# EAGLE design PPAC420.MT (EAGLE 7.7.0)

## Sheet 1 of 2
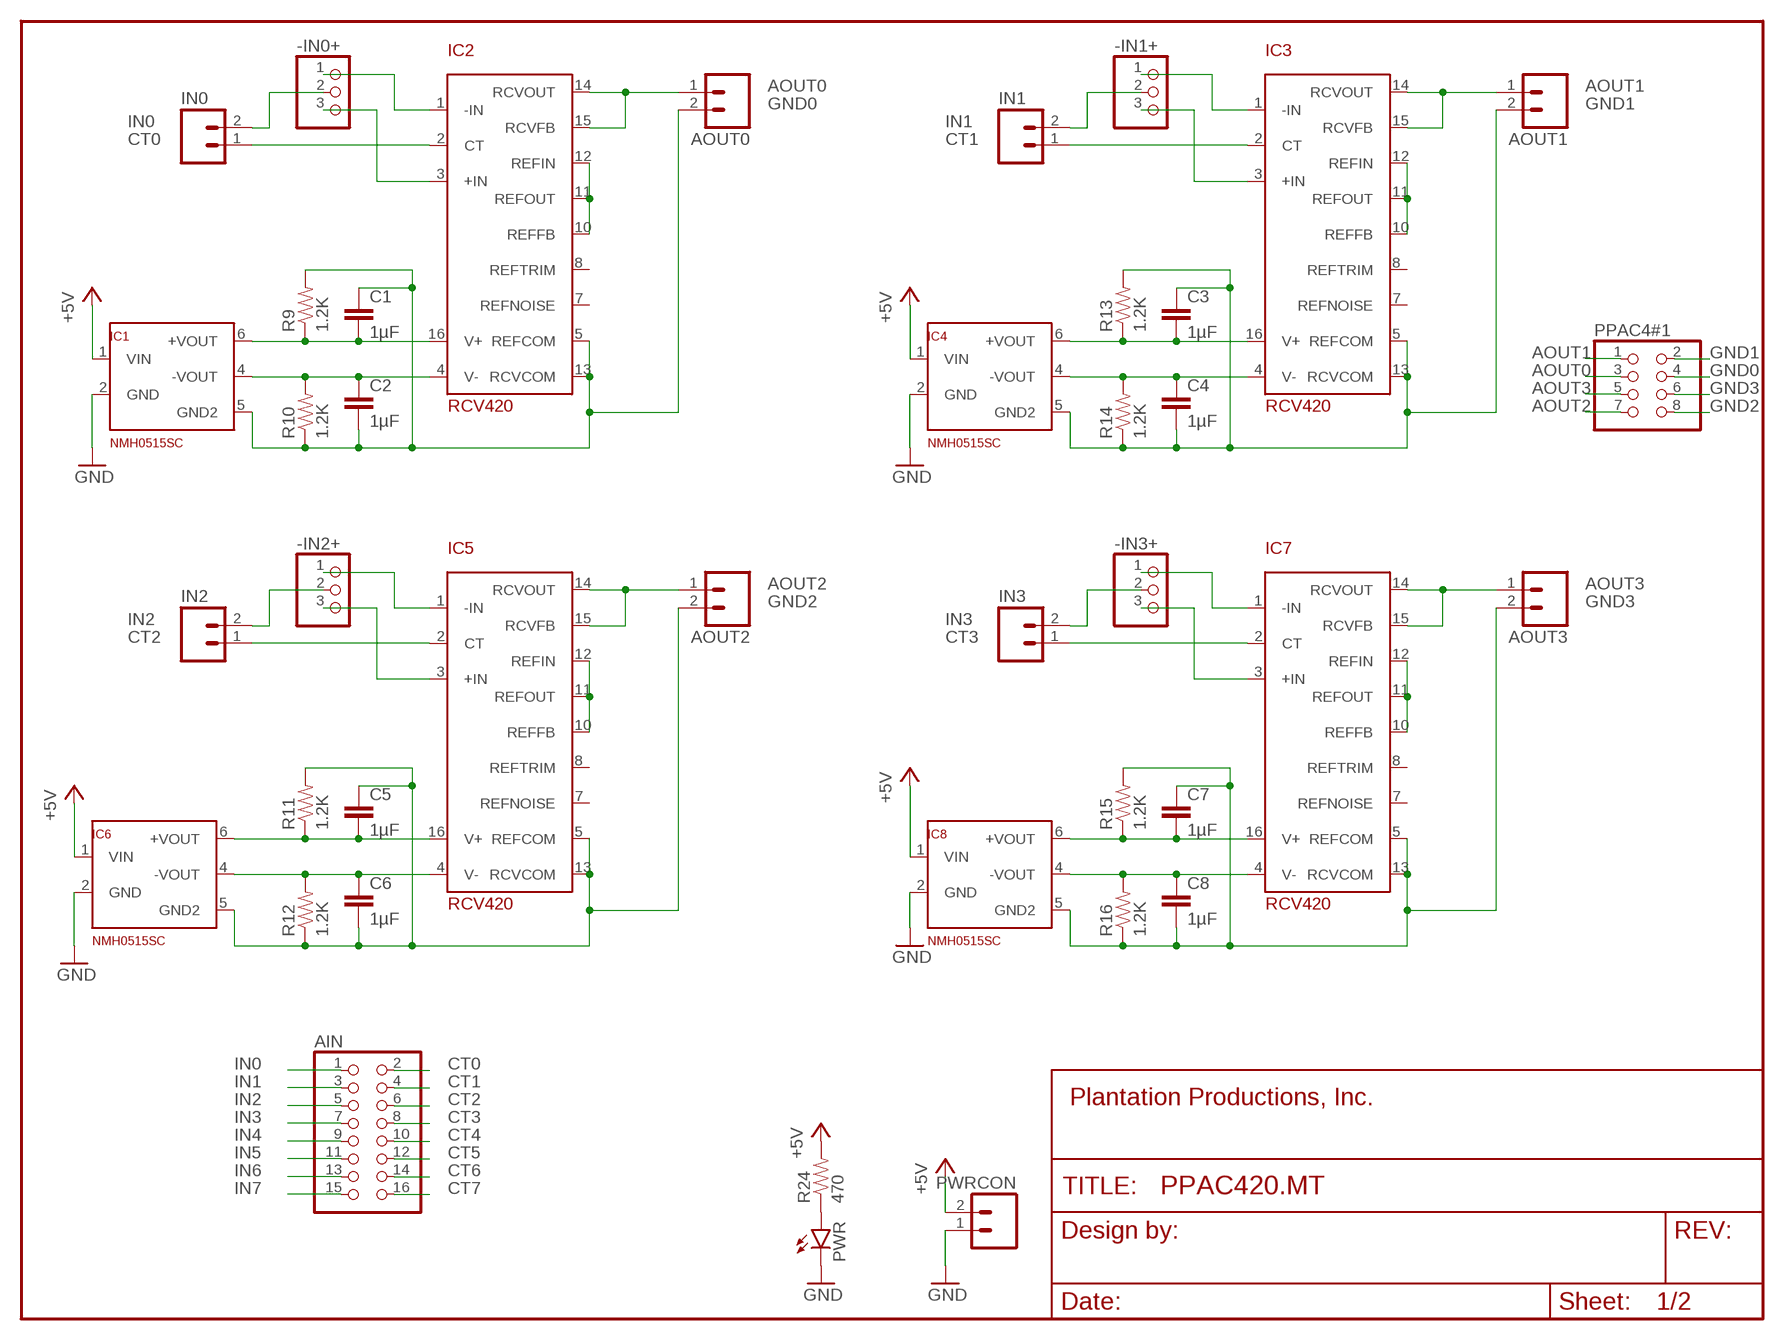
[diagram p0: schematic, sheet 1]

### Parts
-IN0+  PINHD-1X3  [1X03]
-IN1+  PINHD-1X3  [1X03]
-IN2+  PINHD-1X3  [1X03]
-IN3+  PINHD-1X3  [1X03]
AIN  PINHD-2X8  [2X08]
AOUT0  M025MM  [SCREWTERMINAL-5MM-2]
AOUT1  M025MM  [SCREWTERMINAL-5MM-2]
AOUT2  M025MM  [SCREWTERMINAL-5MM-2]
AOUT3  M025MM  [SCREWTERMINAL-5MM-2]
C1  1µF  CAPPTH1  [CAP-PTH-5MM]
C2  1µF  CAPPTH1  [CAP-PTH-5MM]
C3  1µF  CAPPTH1  [CAP-PTH-5MM]
C4  1µF  CAPPTH1  [CAP-PTH-5MM]
C5  1µF  CAPPTH1  [CAP-PTH-5MM]
C6  1µF  CAPPTH1  [CAP-PTH-5MM]
C7  1µF  CAPPTH1  [CAP-PTH-5MM]
C8  1µF  CAPPTH1  [CAP-PTH-5MM]
FRAME4  FRAME-LETTERNO_PACKAGE  [DUMMY]
IC1  NMH0515SC  [SIL6-5A]
IC2  RCV420  [DIL16]
IC3  RCV420  [DIL16]
IC4  NMH0515SC  [SIL6-5A]
IC5  RCV420  [DIL16]
IC6  NMH0515SC  [SIL6-5A]
IC7  RCV420  [DIL16]
IC8  NMH0515SC  [SIL6-5A]
IN0  M025MM  [SCREWTERMINAL-5MM-2]
IN1  M025MM  [SCREWTERMINAL-5MM-2]
IN2  M025MM  [SCREWTERMINAL-5MM-2]
IN3  M025MM  [SCREWTERMINAL-5MM-2]
PPAC4#1  PINHD-2X4  [2X04]
PWR  LED5MM  [LED5MM]
PWRCON  M025MM  [SCREWTERMINAL-5MM-2]
R9  1.2K  1KOHM-1/4W-1%(PTH)  [AXIAL-0.3]
R10  1.2K  1KOHM-1/4W-1%(PTH)  [AXIAL-0.3]
R11  1.2K  1KOHM-1/4W-1%(PTH)  [AXIAL-0.3]
R12  1.2K  1KOHM-1/4W-1%(PTH)  [AXIAL-0.3]
R13  1.2K  1KOHM-1/4W-1%(PTH)  [AXIAL-0.3]
R14  1.2K  1KOHM-1/4W-1%(PTH)  [AXIAL-0.3]
R15  1.2K  1KOHM-1/4W-1%(PTH)  [AXIAL-0.3]
R16  1.2K  1KOHM-1/4W-1%(PTH)  [AXIAL-0.3]
R24  470  1KOHM-1/4W-1%(PTH)  [AXIAL-0.3]

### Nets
+5V: IC1.1(VIN) IC4.1(VIN) IC6.1(VIN) IC8.1(VIN) PWRCON.2 R24.P$2 ; also sheet 2
+15_0: C1.2 IC1.6(+VOUT) IC2.16(V+) R9.P$1
+15_1: C3.2 IC3.16(V+) IC4.6(+VOUT) R13.P$1
+15_2: C5.2 IC5.16(V+) IC6.6(+VOUT) R11.P$1
+15_3: C7.2 IC7.16(V+) IC8.6(+VOUT) R15.P$1
-15_0: C2.1 IC1.4(-VOUT) IC2.4(V-) R10.P$2
-15_1: C4.1 IC3.4(V-) IC4.4(-VOUT) R14.P$2
-15_2: C6.1 IC5.4(V-) IC6.4(-VOUT) R12.P$2
-15_3: C8.1 IC7.4(V-) IC8.4(-VOUT) R16.P$2
AOUT0: AOUT0.1 IC2.14(RCVOUT) IC2.15(RCVFB) PPAC4#1.3
AOUT1: AOUT1.1 IC3.14(RCVOUT) IC3.15(RCVFB) PPAC4#1.1
AOUT2: AOUT2.1 IC5.14(RCVOUT) IC5.15(RCVFB) PPAC4#1.7
AOUT3: AOUT3.1 IC7.14(RCVOUT) IC7.15(RCVFB) PPAC4#1.5
CT0: AIN.2 IC2.2(CT) IN0.1
CT1: AIN.4 IC3.2(CT) IN1.1
CT2: AIN.6 IC5.2(CT) IN2.1
CT3: AIN.8 IC7.2(CT) IN3.1
CT4: AIN.10 ; also sheet 2
CT5: AIN.12 ; also sheet 2
CT6: AIN.14 ; also sheet 2
CT7: AIN.16 ; also sheet 2
GND [Ground]: IC1.2(GND) IC4.2(GND) IC6.2(GND) IC8.2(GND) PWR.K(C) PWRCON.1 ; also sheet 2
GND0 [Ground]: AOUT0.2 C1.1 C2.2 IC1.5(GND2) IC2.5(REFCOM) IC2.13(RCVCOM) PPAC4#1.4 R9.P$2 R10.P$1
GND1: AOUT1.2 C3.1 C4.2 IC3.5(REFCOM) IC3.13(RCVCOM) IC4.5(GND2) PPAC4#1.2 R13.P$2 R14.P$1
GND2: AOUT2.2 C5.1 C6.2 IC5.5(REFCOM) IC5.13(RCVCOM) IC6.5(GND2) PPAC4#1.8 R11.P$2 R12.P$1
GND3: AOUT3.2 C7.1 C8.2 IC7.5(REFCOM) IC7.13(RCVCOM) IC8.5(GND2) PPAC4#1.6 R15.P$2 R16.P$1
IN0: -IN0+.2 AIN.1 IN0.2
IN1: -IN1+.2 AIN.3 IN1.2
IN2: -IN2+.2 AIN.5 IN2.2
IN3: -IN3+.2 AIN.7 IN3.2
IN4: AIN.9 ; also sheet 2
IN5: AIN.11 ; also sheet 2
IN6: AIN.13 ; also sheet 2
IN7: AIN.15 ; also sheet 2
N$3: IC2.10(REFFB) IC2.11(REFOUT) IC2.12(REFIN)
N$4: IC3.10(REFFB) IC3.11(REFOUT) IC3.12(REFIN)
N$7: IC5.10(REFFB) IC5.11(REFOUT) IC5.12(REFIN)
N$10: IC7.10(REFFB) IC7.11(REFOUT) IC7.12(REFIN)
N$25: -IN1+.1 IC3.1(-IN)
N$26: -IN1+.3 IC3.3(+IN)
N$27: -IN0+.1 IC2.1(-IN)
N$28: -IN0+.3 IC2.3(+IN)
N$29: -IN2+.1 IC5.1(-IN)
N$30: -IN2+.3 IC5.3(+IN)
N$31: -IN3+.1 IC7.1(-IN)
N$32: -IN3+.3 IC7.3(+IN)
N$41: PWR.A R24.P$1
Unconnected: IC2.6(NCA) IC2.7(REFNOISE) IC2.8(REFTRIM) IC2.9(NCB) IC3.6(NCA) IC3.7(REFNOISE) IC3.8(REFTRIM) IC3.9(NCB) IC5.6(NCA) IC5.7(REFNOISE) IC5.8(REFTRIM) IC5.9(NCB) IC7.6(NCA) IC7.7(REFNOISE) IC7.8(REFTRIM) IC7.9(NCB)

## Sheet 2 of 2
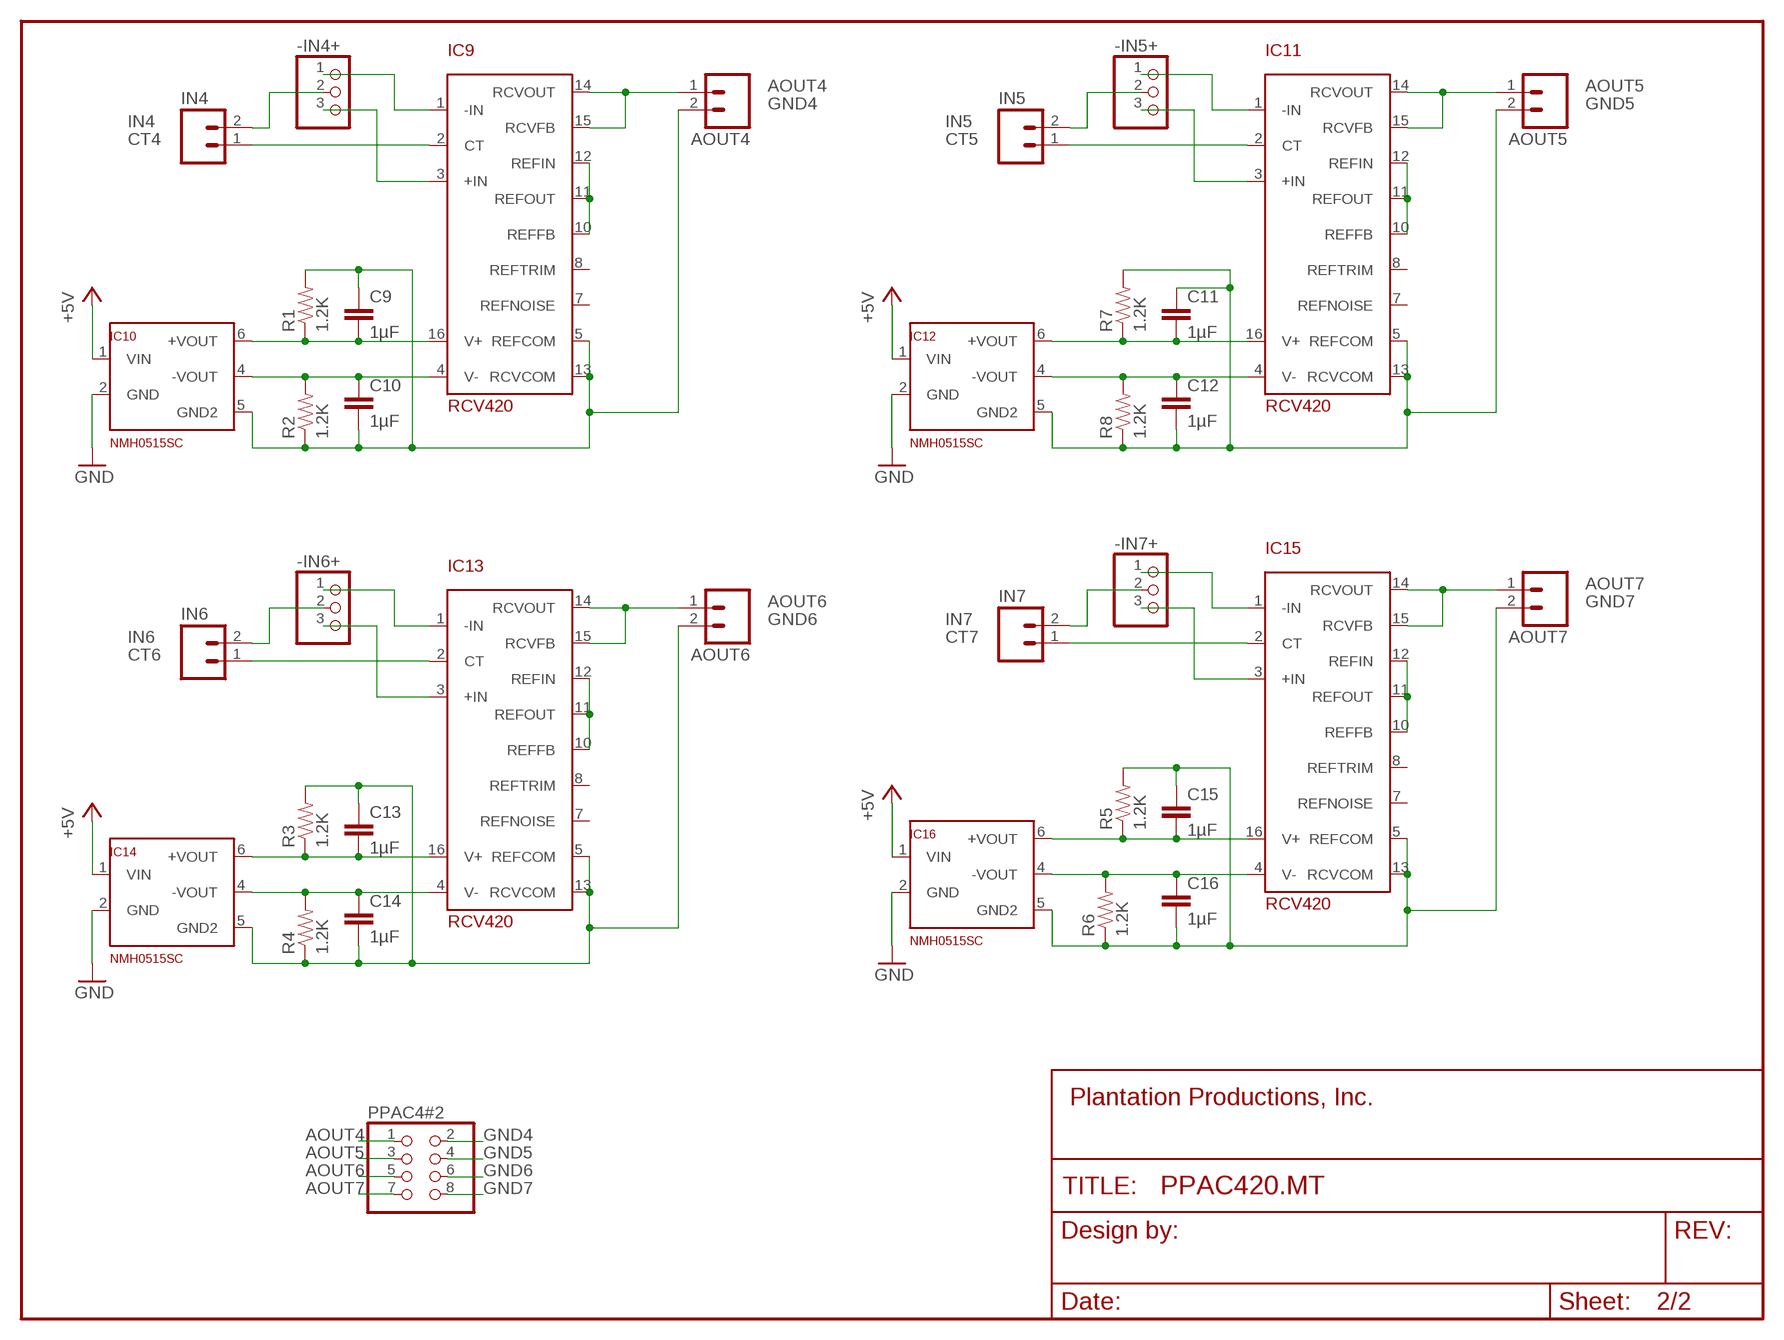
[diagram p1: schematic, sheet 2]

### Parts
-IN4+  PINHD-1X3  [1X03]
-IN5+  PINHD-1X3  [1X03]
-IN6+  PINHD-1X3  [1X03]
-IN7+  PINHD-1X3  [1X03]
AOUT4  M025MM  [SCREWTERMINAL-5MM-2]
AOUT5  M025MM  [SCREWTERMINAL-5MM-2]
AOUT6  M025MM  [SCREWTERMINAL-5MM-2]
AOUT7  M025MM  [SCREWTERMINAL-5MM-2]
C9  1µF  CAPPTH1  [CAP-PTH-5MM]
C10  1µF  CAPPTH1  [CAP-PTH-5MM]
C11  1µF  CAPPTH1  [CAP-PTH-5MM]
C12  1µF  CAPPTH1  [CAP-PTH-5MM]
C13  1µF  CAPPTH1  [CAP-PTH-5MM]
C14  1µF  CAPPTH1  [CAP-PTH-5MM]
C15  1µF  CAPPTH1  [CAP-PTH-5MM]
C16  1µF  CAPPTH1  [CAP-PTH-5MM]
FRAME1  FRAME-LETTERNO_PACKAGE  [DUMMY]
IC9  RCV420  [DIL16]
IC10  NMH0515SC  [SIL6-5A]
IC11  RCV420  [DIL16]
IC12  NMH0515SC  [SIL6-5A]
IC13  RCV420  [DIL16]
IC14  NMH0515SC  [SIL6-5A]
IC15  RCV420  [DIL16]
IC16  NMH0515SC  [SIL6-5A]
IN4  M025MM  [SCREWTERMINAL-5MM-2]
IN5  M025MM  [SCREWTERMINAL-5MM-2]
IN6  M025MM  [SCREWTERMINAL-5MM-2]
IN7  M025MM  [SCREWTERMINAL-5MM-2]
PPAC4#2  PINHD-2X4  [2X04]
R1  1.2K  1KOHM-1/4W-1%(PTH)  [AXIAL-0.3]
R2  1.2K  1KOHM-1/4W-1%(PTH)  [AXIAL-0.3]
R3  1.2K  1KOHM-1/4W-1%(PTH)  [AXIAL-0.3]
R4  1.2K  1KOHM-1/4W-1%(PTH)  [AXIAL-0.3]
R5  1.2K  1KOHM-1/4W-1%(PTH)  [AXIAL-0.3]
R6  1.2K  1KOHM-1/4W-1%(PTH)  [AXIAL-0.3]
R7  1.2K  1KOHM-1/4W-1%(PTH)  [AXIAL-0.3]
R8  1.2K  1KOHM-1/4W-1%(PTH)  [AXIAL-0.3]

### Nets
+5V: IC10.1(VIN) IC12.1(VIN) IC14.1(VIN) IC16.1(VIN) ; also sheet 1
+15_4: C9.2 IC9.16(V+) IC10.6(+VOUT) R1.P$1
+15_5: C11.2 IC11.16(V+) IC12.6(+VOUT) R7.P$1
+15_6: C13.2 IC13.16(V+) IC14.6(+VOUT) R3.P$1
+15_7: C15.2 IC15.16(V+) IC16.6(+VOUT) R5.P$1
-15_4: C10.1 IC9.4(V-) IC10.4(-VOUT) R2.P$2
-15_5: C12.1 IC11.4(V-) IC12.4(-VOUT) R8.P$2
-15_6: C14.1 IC13.4(V-) IC14.4(-VOUT) R4.P$2
-15_7: C16.1 IC15.4(V-) IC16.4(-VOUT) R6.P$2
AOUT4: AOUT4.1 IC9.14(RCVOUT) IC9.15(RCVFB) PPAC4#2.1
AOUT5: AOUT5.1 IC11.14(RCVOUT) IC11.15(RCVFB) PPAC4#2.3
AOUT6: AOUT6.1 IC13.14(RCVOUT) IC13.15(RCVFB) PPAC4#2.5
AOUT7: AOUT7.1 IC15.14(RCVOUT) IC15.15(RCVFB) PPAC4#2.7
CT4: IC9.2(CT) IN4.1 ; also sheet 1
CT5: IC11.2(CT) IN5.1 ; also sheet 1
CT6: IC13.2(CT) IN6.1 ; also sheet 1
CT7: IC15.2(CT) IN7.1 ; also sheet 1
GND [Ground]: IC10.2(GND) IC12.2(GND) IC14.2(GND) IC16.2(GND) ; also sheet 1
GND4: AOUT4.2 C9.1 C10.2 IC9.5(REFCOM) IC9.13(RCVCOM) IC10.5(GND2) PPAC4#2.2 R1.P$2 R2.P$1
GND5: AOUT5.2 C11.1 C12.2 IC11.5(REFCOM) IC11.13(RCVCOM) IC12.5(GND2) PPAC4#2.4 R7.P$2 R8.P$1
GND6: AOUT6.2 C13.1 C14.2 IC13.5(REFCOM) IC13.13(RCVCOM) IC14.5(GND2) PPAC4#2.6 R3.P$2 R4.P$1
GND7: AOUT7.2 C15.1 C16.2 IC15.5(REFCOM) IC15.13(RCVCOM) IC16.5(GND2) PPAC4#2.8 R5.P$2 R6.P$1
IN4: -IN4+.2 IN4.2 ; also sheet 1
IN5: -IN5+.2 IN5.2 ; also sheet 1
IN6: -IN6+.2 IN6.2 ; also sheet 1
IN7: -IN7+.2 IN7.2 ; also sheet 1
N$13: IC9.10(REFFB) IC9.11(REFOUT) IC9.12(REFIN)
N$16: IC11.10(REFFB) IC11.11(REFOUT) IC11.12(REFIN)
N$19: IC13.10(REFFB) IC13.11(REFOUT) IC13.12(REFIN)
N$22: IC15.10(REFFB) IC15.11(REFOUT) IC15.12(REFIN)
N$33: -IN4+.1 IC9.1(-IN)
N$34: -IN4+.3 IC9.3(+IN)
N$35: -IN5+.1 IC11.1(-IN)
N$36: -IN5+.3 IC11.3(+IN)
N$37: -IN6+.1 IC13.1(-IN)
N$38: -IN6+.3 IC13.3(+IN)
N$39: -IN7+.1 IC15.1(-IN)
N$40: -IN7+.3 IC15.3(+IN)
Unconnected: IC9.6(NCA) IC9.7(REFNOISE) IC9.8(REFTRIM) IC9.9(NCB) IC11.6(NCA) IC11.7(REFNOISE) IC11.8(REFTRIM) IC11.9(NCB) IC13.6(NCA) IC13.7(REFNOISE) IC13.8(REFTRIM) IC13.9(NCB) IC15.6(NCA) IC15.7(REFNOISE) IC15.8(REFTRIM) IC15.9(NCB)

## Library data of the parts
-IN0+ -IN1+ -IN2+ -IN3+ -IN4+ -IN5+ -IN6+ -IN7+ = pinhead:PINHD-1X3: PIN HEADER
AIN = pinhead:PINHD-2X8: PIN HEADER
AOUT0 AOUT1-AOUT7 IN0 IN1-IN7 PWRCON = SparkFun-Connectors:M02: Standard 2-pin 0.1" header. Use with; STOREFRONT_ID: PRT-08432
C1-C16 = SparkFun-Passives:CAP: Capacitor
FRAME1 FRAME4 = SparkFun-Aesthetics:FRAME-LETTER: Schematic Frame; DESIGNER: Nobody; VERSION: v01
IC1 IC4 IC6 IC8 IC10 IC12 IC14 IC16 = PlantProd:NMH0515SC: NMH0515 Isolated Power Supply 5V to +/-15V
IC2 IC3 IC5 IC7 IC9 IC11 IC13 IC15 = PlantProd:RCV420: RCV420 4-20ma receiver
PPAC4#1 PPAC4#2 = pinhead:PINHD-2X4: PIN HEADER
PWR = SparkFun-LED:LED: LEDs
R1-R16 R24 = SparkFun-Resistors:1KOHM-1/4W-1%(PTH): RES-12182; PROD_ID: RES-12182; VALUE: 1K

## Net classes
1 Ground: width 0.762 mm, drill 1 mm, clearance 0.102 mm
2 RelayConn: width 1.016 mm, drill 0.025 mm, clearance 0.508 mm
3 HiCurSignal: width 1.016 mm, drill 0.025 mm, clearance 1.016 mm

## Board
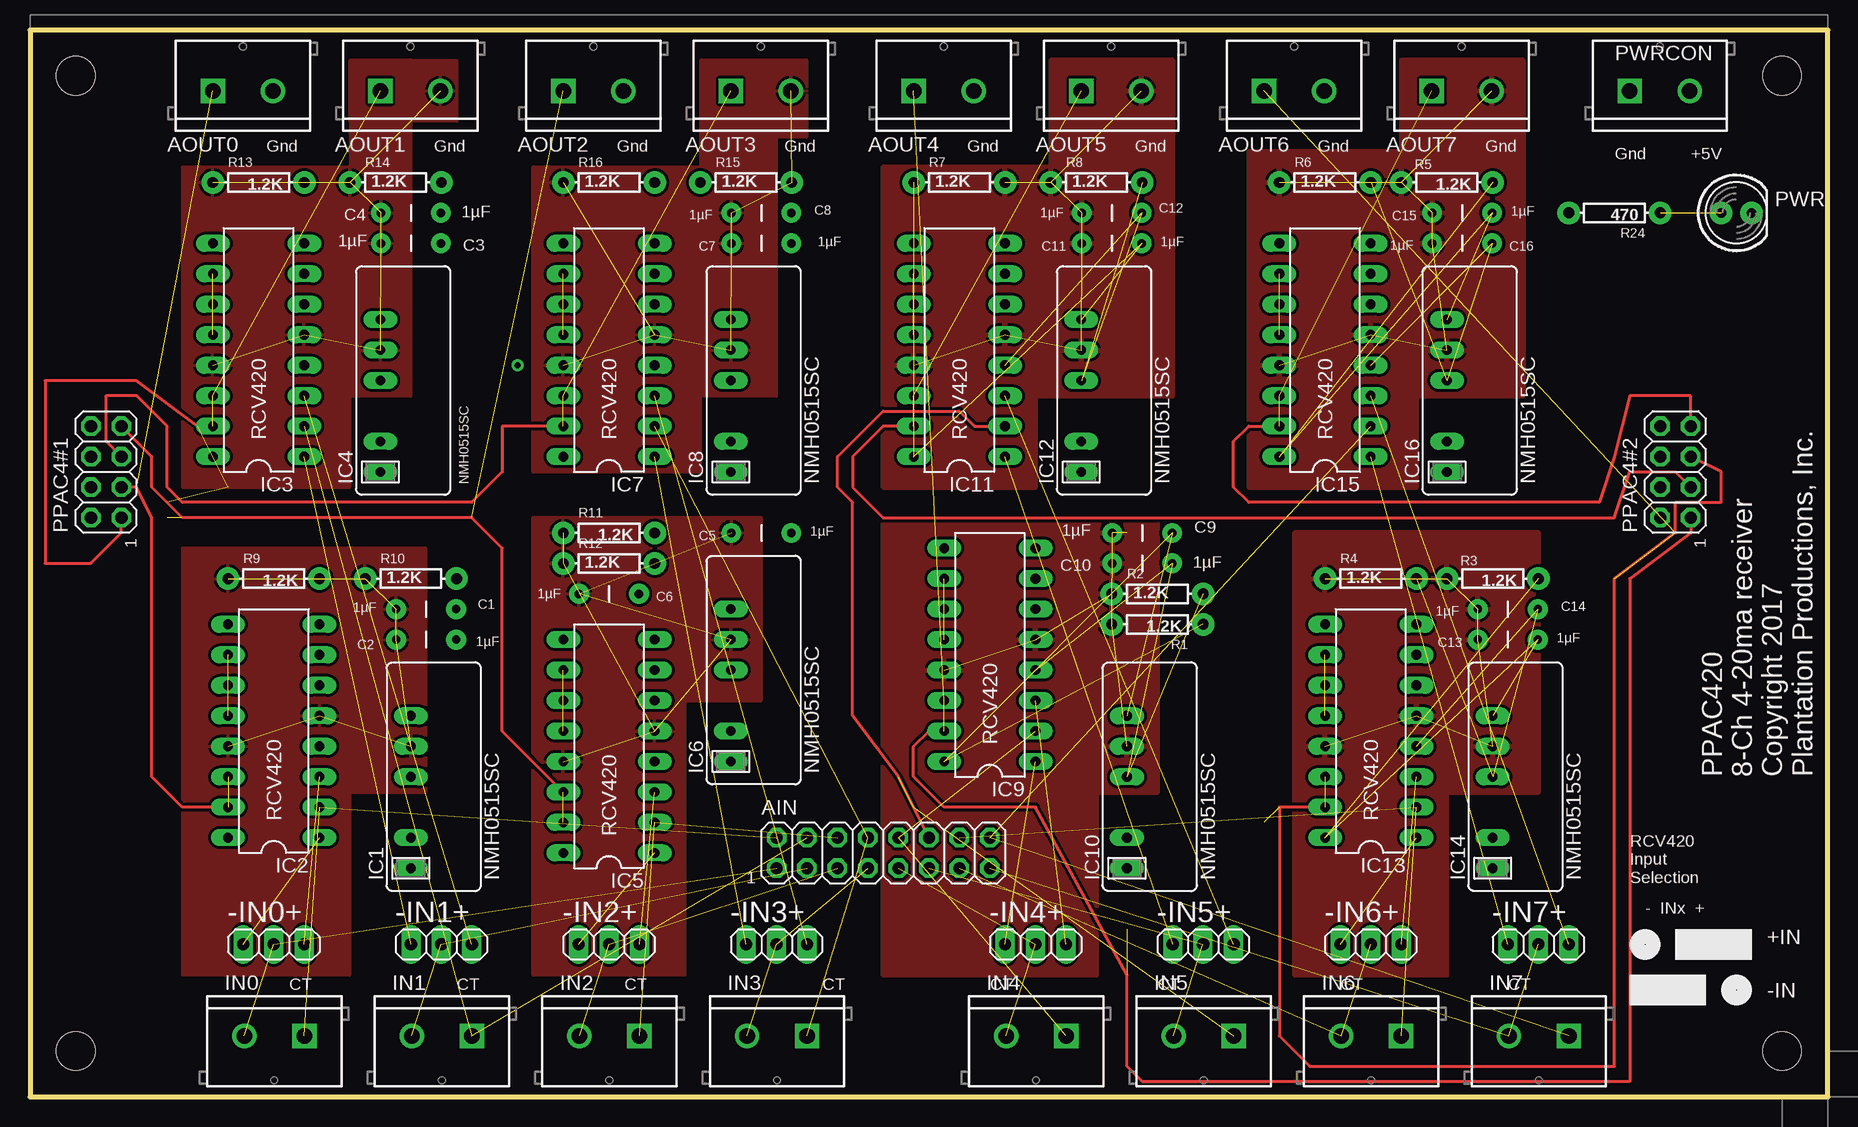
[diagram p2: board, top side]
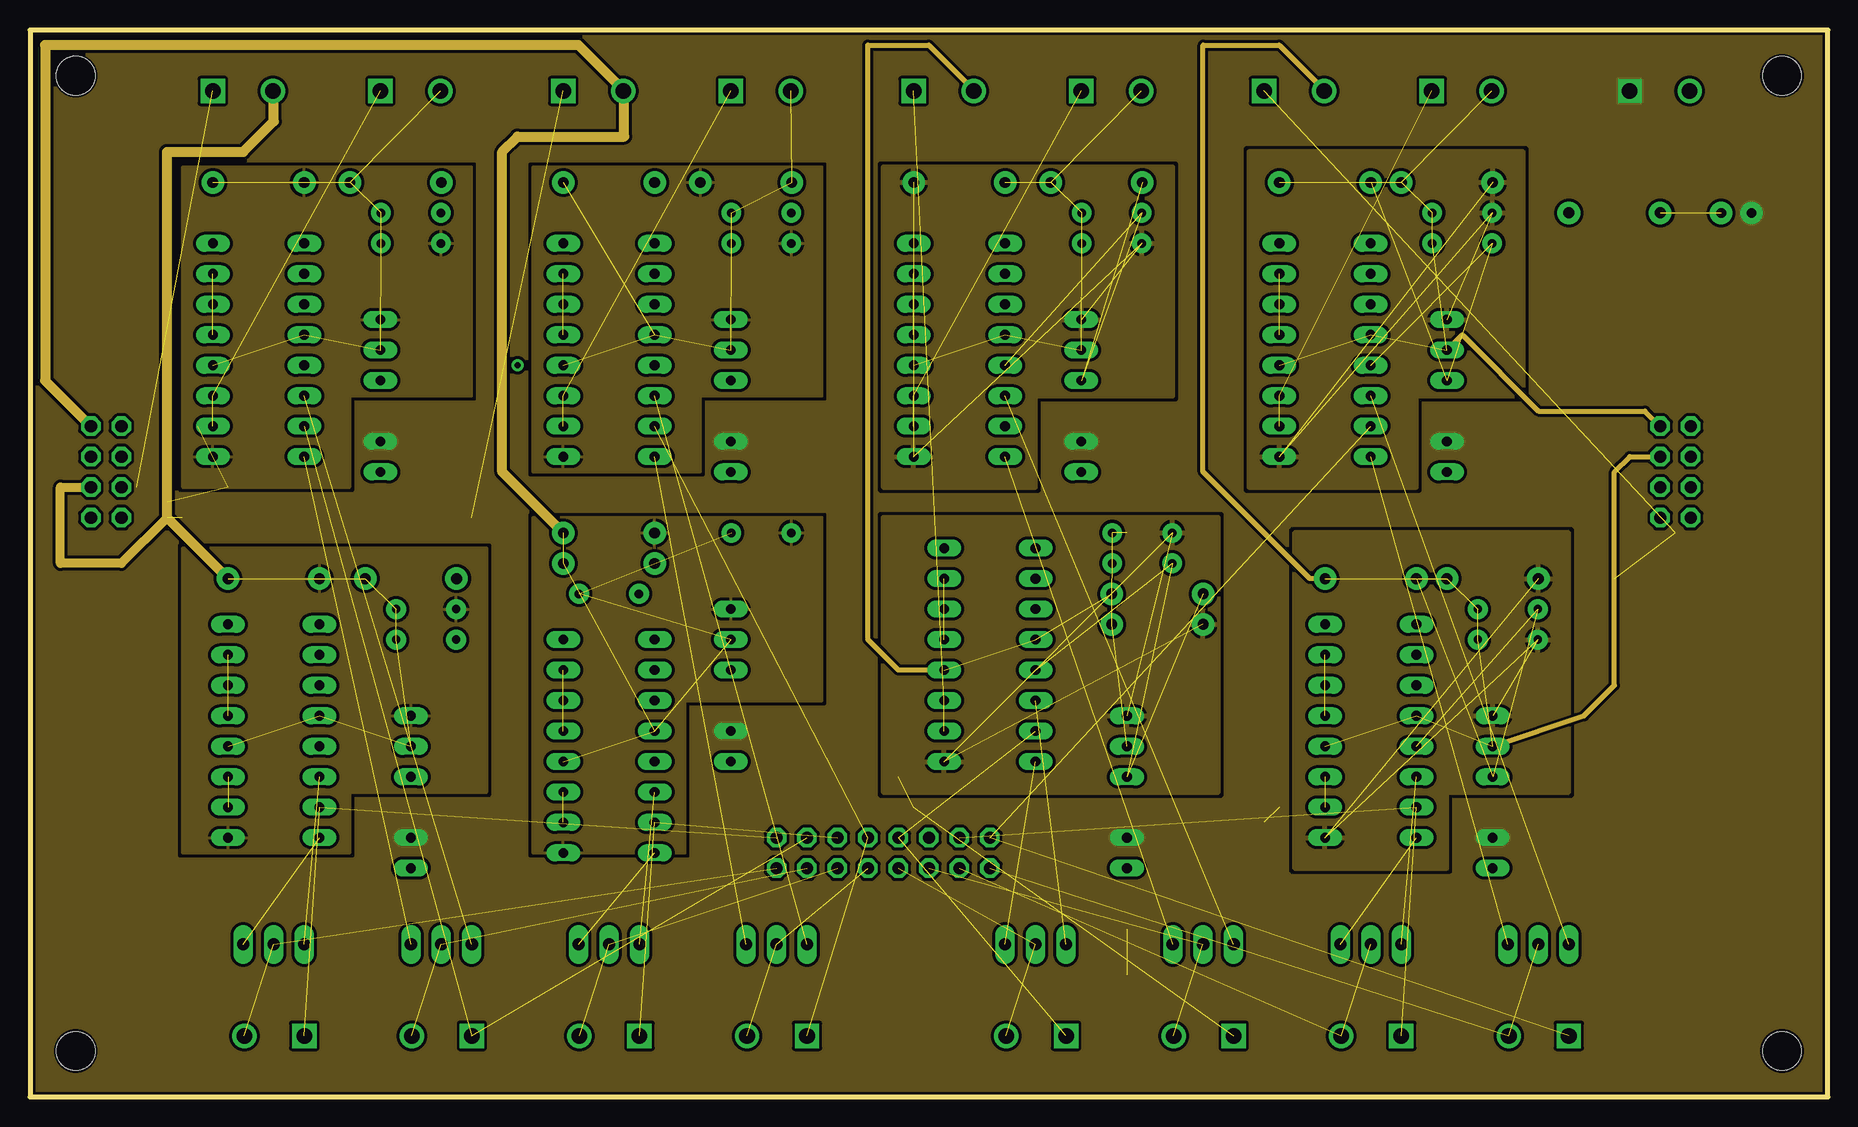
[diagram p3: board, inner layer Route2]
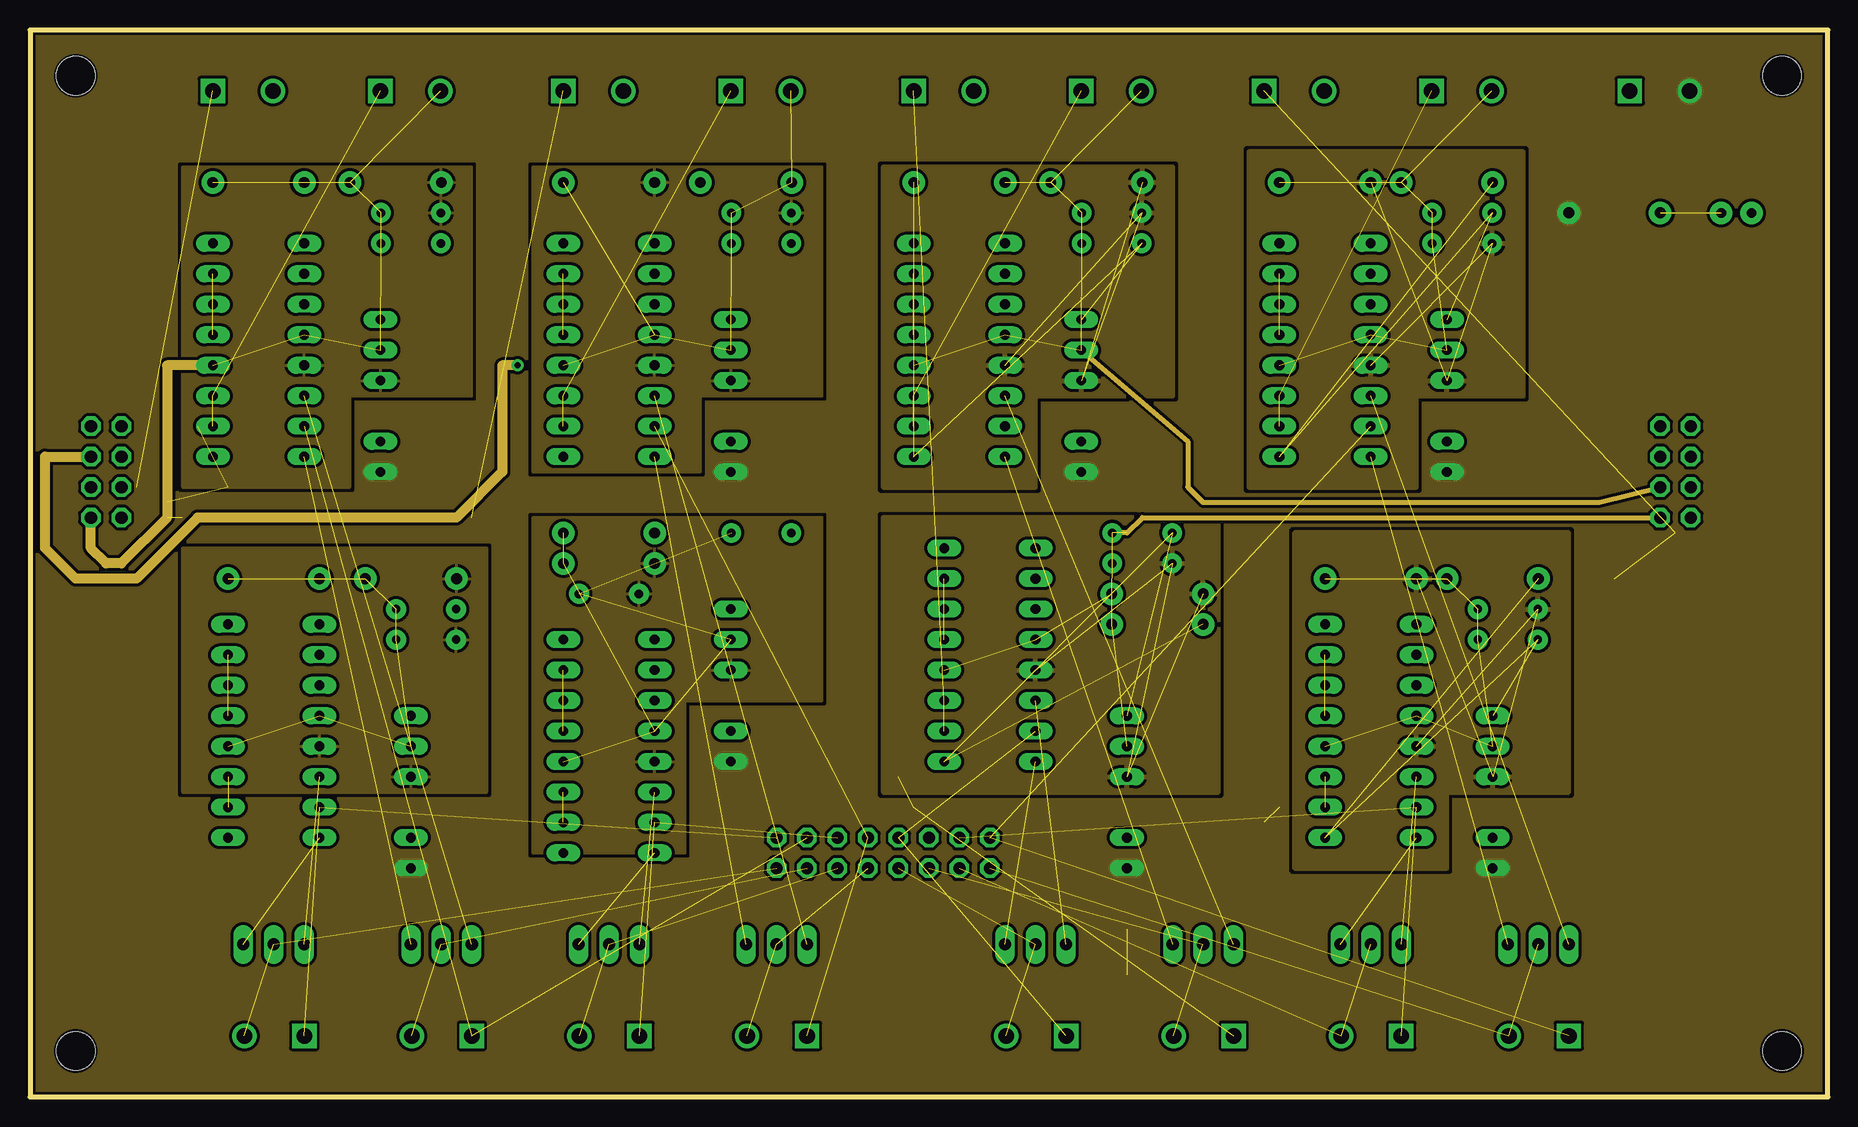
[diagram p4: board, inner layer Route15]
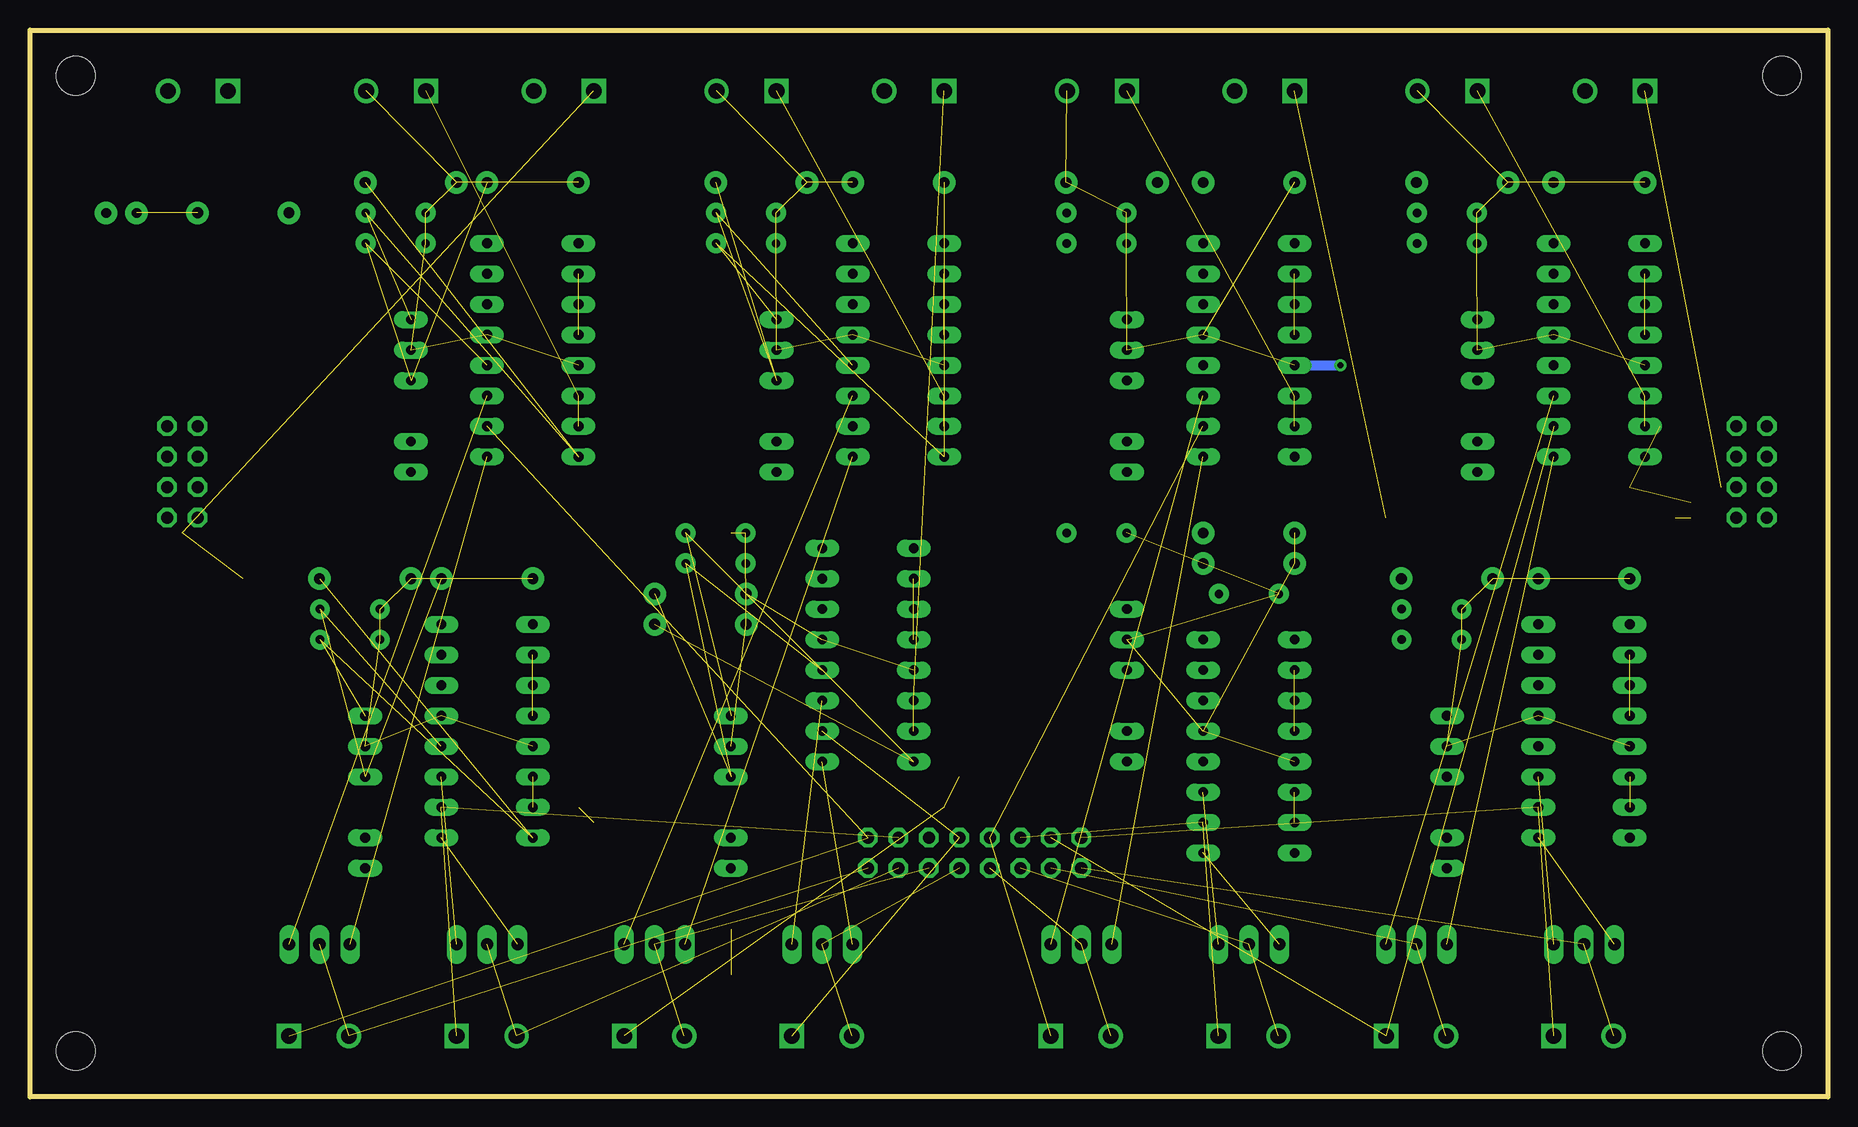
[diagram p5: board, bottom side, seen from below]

Size 149.86 x 88.9 mm. Coordinates in mm from the lower left corner, seen from the top.
Outline: 0,0 149.86,0 149.86,88.9 0,88.9 0,0
Copper layers (1*2*15*16): Top 0.035mm / dielectric 1.5mm / Route2 0.035mm / dielectric 0.15mm / Route15 0.035mm / dielectric 0.2mm / Bottom 0.035mm
Design rules "SeeedStudio_2layer_DRU_no_angle_20140221 *": minimum track width 10mil, minimum drill 20mil, track to track 10mil, track to pad 10mil, pad to pad 10mil, via to via 10mil, smd to smd 8mil, copper to edge 8mil, drill to drill 8mil, minimum pad ring 12mil, minimum via ring 10mil, stop-mask expansion 4mil, vias tented up to drill 25mil, thermal gap 10mil
Holes 3.2 mm at 3.81,85.09 3.81,3.81 146.05,85.09 146.05,3.81

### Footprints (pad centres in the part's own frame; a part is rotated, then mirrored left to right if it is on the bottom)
1X03 = drill 1.016 long: 1 -2.54,0; 2 0,0; 3 2.54,0
2X08 = drill 1.016 octagon: 1 -8.89,-1.27; 2 -8.89,1.27; 3 -6.35,-1.27; 4 -6.35,1.27; 5 -3.81,-1.27; 6 -3.81,1.27; 7 -1.27,-1.27; 8 -1.27,1.27; 9 1.27,-1.27; 10 1.27,1.27; 11 3.81,-1.27; 12 3.81,1.27; 13 6.35,-1.27; 14 6.35,1.27; 15 8.89,-1.27; 16 8.89,1.27
SCREWTERMINAL-5MM-2 = drill 1.3 pad 2.032 square: 1 0,0 | drill 1.3 pad 2.032: 2 5,0
CAP-PTH-5MM = drill 0.7 pad 1.651: 1 -2.5,0; 2 2.5,0
SIL6-5A = drill 0.813 long: 1 -5.08,0; 2 -2.54,0; 4 2.54,0; 5 5.08,0; 6 7.62,0
DIL16 = drill 0.813 long: 1 -8.89,-3.81; 2 -6.35,-3.81; 3 -3.81,-3.81; 4 -1.27,-3.81; 5 1.27,-3.81; 6 3.81,-3.81; 7 6.35,-3.81; 8 8.89,-3.81; 9 8.89,3.81; 10 6.35,3.81; 11 3.81,3.81; 12 1.27,3.81; 13 -1.27,3.81; 14 -3.81,3.81; 15 -6.35,3.81; 16 -8.89,3.81
2X04 = drill 1.016 octagon: 1 -3.81,-1.27; 2 -3.81,1.27; 3 -1.27,-1.27; 4 -1.27,1.27; 5 1.27,-1.27; 6 1.27,1.27; 7 3.81,-1.27; 8 3.81,1.27
LED5MM = drill 0.813 pad 1.88: A -1.27,0; K 1.27,0
AXIAL-0.3 = drill 0.9 pad 1.88: P$1 -3.81,0; P$2 3.81,0

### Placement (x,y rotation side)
-IN0+  20.32,12.7 0 top
-IN1+  34.29,12.7 0 top
-IN2+  48.26,12.7 0 top
-IN3+  62.23,12.7 0 top
-IN4+  83.82,12.7 0 top
-IN5+  97.79,12.7 0 top
-IN6+  111.76,12.7 0 top
-IN7+  125.73,12.7 0 top
AIN  71.12,20.32 0 top
AOUT0  15.24,83.82 0 top
AOUT1  29.21,83.82 0 top
AOUT2  44.45,83.82 0 top
AOUT3  58.42,83.82 0 top
AOUT4  73.66,83.82 0 top
AOUT5  87.63,83.82 0 top
AOUT6  102.87,83.82 0 top
AOUT7  116.84,83.82 0 top
C1  33.02,40.64 0 top
C2  33.02,38.1 180 top
C3  31.75,71.12 0 top
C4  31.75,73.66 180 top
C5  60.96,46.99 0 top
C6  48.26,41.91 180 top
C7  60.96,71.12 0 top
C8  60.96,73.66 180 top
C9  92.71,46.99 0 top
C10  92.71,44.45 180 top
C11  90.17,71.12 0 top
C12  90.17,73.66 180 top
C13  123.19,38.1 0 top
C14  123.19,40.64 180 top
C15  119.38,73.66 0 top
C16  119.38,71.12 180 top
FRAME1  not placed on the board
FRAME4  not placed on the board
IC1  31.75,24.13 90 top
IC2  20.32,30.48 90 top
IC3  19.05,62.23 90 top
IC4  29.21,57.15 90 top
IC5  48.26,29.21 90 top
IC6  58.42,33.02 90 top
IC7  48.26,62.23 90 top
IC8  58.42,57.15 90 top
IC9  80.01,36.83 90 top
IC10  91.44,24.13 90 top
IC11  77.47,62.23 90 top
IC12  87.63,57.15 90 top
IC13  111.76,30.48 90 top
IC14  121.92,24.13 90 top
IC15  107.95,62.23 90 top
IC16  118.11,57.15 90 top
IN0  22.86,5.08 180 top
IN1  36.83,5.08 180 top
IN2  50.8,5.08 180 top
IN3  64.77,5.08 180 top
IN4  86.36,5.08 180 top
IN5  100.33,5.08 180 top
IN6  114.3,5.08 180 top
IN7  128.27,5.08 180 top
PPAC4#1  6.35,52.07 90 top
PPAC4#2  137.16,52.07 90 top
PWR  142.24,73.66 0 top
PWRCON  133.35,83.82 0 top
R1  93.98,39.37 180 top
R2  93.98,41.91 0 top
R3  121.92,43.18 180 top
R4  111.76,43.18 0 top
R5  118.11,76.2 180 top
R6  107.95,76.2 0 top
R7  77.47,76.2 0 top
R8  88.9,76.2 0 top
R9  20.32,43.18 180 top
R10  31.75,43.18 0 top
R11  48.26,46.99 180 top
R12  48.26,44.45 0 top
R13  19.05,76.2 180 top
R14  30.48,76.2 0 top
R15  59.69,76.2 0 top
R16  48.26,76.2 0 top
R24  132.08,73.66 180 top

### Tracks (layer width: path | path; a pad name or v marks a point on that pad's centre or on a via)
+5V
  pour Route15 (rank 2, no thermals): 0,88.9 149.86,88.9 149.86,0 0,0
+15_0
  pour Route2: 12.7,20.32 26.67,20.32 26.67,25.4 38.1,25.4 38.1,45.72 12.7,45.72
+15_1
  pour Route2: 12.7,50.8 26.67,50.8 26.67,58.42 36.83,58.42 36.83,77.47 12.7,77.47
+15_2
  pour Route2 (rank 2): 41.91,20.32 54.61,20.32 54.61,33.02 66.04,33.02 66.04,48.26 41.91,48.26
+15_3
  pour Route2: 41.91,52.07 55.88,52.07 55.88,58.42 66.04,58.42 66.04,77.47 41.91,77.47
+15_4  (3 unrouted)
  pour Route2: 71.12,25.4 99.06,25.4 99.06,48.26 71.12,48.26
+15_5  (3 unrouted)
  pour Route2: 71.12,50.8 83.82,50.8 83.82,58.42 95.25,58.42 95.25,77.47 71.12,77.47
+15_6  (3 unrouted)
  pour Route2: 105.41,19.05 118.11,19.05 118.11,25.4 128.27,25.4 128.27,46.99 105.41,46.99
+15_7  (3 unrouted)
  pour Route2: 101.6,50.8 115.57,50.8 115.57,58.42 124.46,58.42 124.46,78.74 101.6,78.74
-15_0
  pour Route15: 12.7,25.4 38.1,25.4 38.1,45.72 12.7,45.72
-15_1
  pour Route15: 12.7,50.8 26.67,50.8 26.67,58.42 36.83,58.42 36.83,77.47 12.7,77.47
-15_2
  pour Route15: 41.91,20.32 54.61,20.32 54.61,33.02 66.04,33.02 66.04,48.26 41.91,48.26
-15_3
  pour Route15: 41.91,52.07 55.88,52.07 55.88,58.42 66.04,58.42 66.04,77.47 41.91,77.47
-15_4  (3 unrouted)
  pour Route15: 71.12,25.4 99.06,25.4 99.06,48.26 71.12,48.26
-15_5  (3 unrouted)
  pour Route15: 71.12,50.8 83.82,50.8 83.82,58.42 95.25,58.42 95.25,77.47 71.12,77.47
-15_6  (3 unrouted)
  pour Route15: 105.41,19.05 118.11,19.05 118.11,25.4 128.27,25.4 128.27,46.99 105.41,46.99
-15_7  (3 unrouted)
  pour Route15: 101.6,50.8 115.57,50.8 115.57,58.42 124.46,58.42 124.46,78.74 101.6,78.74
AOUT0  (2 unrouted)
  Top 0.254: IC2.15 12.7,24.13 10.16,26.67 10.16,48.26 8.89,50.8 PPAC4#1.3
AOUT1  (4 unrouted)
  Top 0.254: IC3.15 13.97,55.88 8.89,59.69 1.27,59.69 1.27,44.45 5.08,44.45 7.62,46.99 PPAC4#1.1
AOUT2  (3 unrouted)
  Top 0.254: IC5.14 39.37,30.48 39.37,45.72 36.83,48.26 12.7,48.26 10.16,50.8 10.16,53.34 PPAC4#1.7
AOUT3  (2 unrouted)
  Top 0.254: IC7.15 39.37,55.88 39.37,52.07 36.83,49.53 12.7,49.53 11.43,50.8 11.43,55.88 8.89,58.42 6.35,58.42 6.35,54.61 PPAC4#1.5
AOUT4  (3 unrouted)
  Top 0.254: PPAC4#2.1 138.43,46.99 133.35,43.18 133.35,1.27 92.71,1.27 91.44,2.54 91.44,10.16 83.82,24.13 76.2,24.13 73.66,26.67 73.66,29.21 74.93,30.48 IC9.15
AOUT5  (2 unrouted)
  Top 0.254: IC11.15 71.12,55.88 68.58,53.34 68.58,50.8 71.12,48.26 132.08,48.26 133.35,52.07 137.16,52.07 PPAC4#2.3
AOUT6  (4 unrouted)
  Top 0.254: IC13.15 104.14,24.13 104.14,5.08 106.68,2.54 132.08,2.54 132.08,43.18 137.16,46.99 137.16,49.53 140.97,49.53 140.97,52.07 PPAC4#2.5
AOUT7  (2 unrouted)
  Top 0.254: PPAC4#2.7 138.43,58.42 133.35,58.42 132.08,53.34 130.81,49.53 101.6,49.53 100.33,50.8 100.33,54.61 101.6,55.88 IC15.15
CT0  (2 unrouted)
CT1  (2 unrouted)
CT2  (2 unrouted)
CT3  (2 unrouted)
CT4  (2 unrouted)
CT5  (2 unrouted)
  Top 0.254: AIN.12 72.39,26.67 68.58,31.75 68.58,49.53 67.31,50.8 67.31,53.34 71.12,57.15 77.47,57.15 78.74,55.88 IC11.2
CT6  (2 unrouted)
CT7  (2 unrouted)
GND
  pour Route2 (rank 6, no thermals): 0,88.9 149.86,88.9 149.86,0 0,0
GND0  (6 unrouted)
  Route2 0.254: 20.32,83.82 AOUT0.2
  Route2 0.762: 11.43,48.26 7.62,44.45 2.54,44.45 2.54,50.8 PPAC4#1.4
  Route2 0.813: R9.P$2 11.43,48.26 11.43,78.74 17.78,78.74 20.32,81.28 20.32,83.82
  pour Top: 12.7,10.16 26.67,10.16 26.67,25.4 33.02,25.4 33.02,45.72 12.7,45.72
GND1  (7 unrouted)
  Route15 0.813: IC3.13 11.43,60.96 11.43,48.26 7.62,44.45 6.35,44.45 5.08,45.72 PPAC4#1.2
  pour Top: 12.7,50.8 26.67,50.8 26.67,58.42 31.75,58.42 31.75,86.36 26.67,86.36 26.67,77.47 12.7,77.47
  pour Top: 26.67,86.36 35.56,86.36 35.56,81.28 26.67,81.28
GND2  (6 unrouted)
  Route2 0.254: 49.53,83.82 AOUT2.2
  Route2 0.813: R11.P$2 39.37,52.07 39.37,78.74 40.64,80.01 49.53,80.01 49.53,83.82 45.72,87.63 1.27,87.63 1.27,59.69 PPAC4#1.8
  pour Top: 43.18,10.16 54.61,10.16 54.61,33.02 60.96,33.02 60.96,48.26 41.91,48.26 41.91,10.16
GND3  (via drill 0.51)  (7 unrouted)
  Route15 0.813: v40.64,60.96 39.37,60.96 39.37,52.07 35.56,48.26 13.97,48.26 8.89,43.18 3.81,43.18 1.27,45.72 1.27,53.34 PPAC4#1.6
  Bottom 0.813: IC7.13 v40.64,60.96
  pour Top: 41.91,52.07 55.88,52.07 55.88,58.42 62.23,58.42 62.23,80.01 64.77,80.01 64.77,86.36 55.88,86.36 55.88,77.47 41.91,77.47
GND4  (7 unrouted)
  Route2 0.406: IC9.13 72.39,35.56 69.85,38.1 69.85,87.63 74.93,87.63 78.74,83.82 AOUT4.2
  Route15 0.406: C9.1 91.44,46.99 92.71,48.26 PPAC4#2.2
  pour Top: 71.12,48.26 71.12,10.16 88.9,10.16 88.9,25.4 93.98,25.4 93.98,48.26
GND5  (7 unrouted)
  Route15 0.406: IC12.5 96.52,54.61 96.52,50.8 97.79,49.53 130.81,49.53 PPAC4#2.4
  pour Top: 72.39,50.8 83.82,50.8 83.82,58.42 95.25,58.42 95.25,86.36 85.09,86.36 85.09,77.47 71.12,77.47 71.12,50.8
GND6  (6 unrouted)
  Route2 0.406: IC14.5 129.54,31.75 132.08,34.29 132.08,52.07 133.35,53.34 PPAC4#2.6 | R4.P$1 106.68,43.18 97.79,52.07 97.79,87.63 104.14,87.63 107.95,83.82 AOUT6.2
  pour Top: 105.41,10.16 118.11,10.16 118.11,25.4 125.73,25.4 125.73,46.99 105.41,46.99
GND7  (7 unrouted)
  Route2 0.406: PPAC4#2.8 134.62,57.15 125.73,57.15 119.38,63.5 IC16.5
  pour Top: 102.87,50.8 115.57,50.8 115.57,58.42 124.46,58.42 124.46,86.36 114.3,86.36 114.3,78.74 101.6,78.74 101.6,50.8
IN0  (2 unrouted)
IN1  (2 unrouted)
IN2  (2 unrouted)
IN3  (2 unrouted)
IN4  (2 unrouted)
IN5  (2 unrouted)
IN6  (2 unrouted)
IN7  (2 unrouted)
N$3  (2 unrouted)
N$4  (2 unrouted)
N$7  (2 unrouted)
N$10  (2 unrouted)
N$13  (2 unrouted)
N$16  (2 unrouted)
N$19  (2 unrouted)
N$22  (2 unrouted)
N$25  (1 unrouted)
N$26  (1 unrouted)
N$27  (1 unrouted)
N$28  (1 unrouted)
N$29  (1 unrouted)
N$30  (1 unrouted)
N$31  (1 unrouted)
N$32  (1 unrouted)
N$33  (1 unrouted)
N$34  (1 unrouted)
N$35  (1 unrouted)
N$36  (1 unrouted)
N$37  (1 unrouted)
N$38  (1 unrouted)
N$39  (1 unrouted)
N$40  (1 unrouted)
N$41  (1 unrouted)

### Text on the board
tPlace: Gnd | Gnd | Gnd | Gnd | Gnd | Gnd | Gnd | Gnd | Gnd | +5V | 1 | 1 | PPAC420 / 8-Ch 4-20ma receiver / Copyright 2017 / Plantation Productions, Inc. | 1 | RCV420 / Input / Selection | - INx + | +IN | CT | CT | CT | CT | CT | CT | CT | CT | -IN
